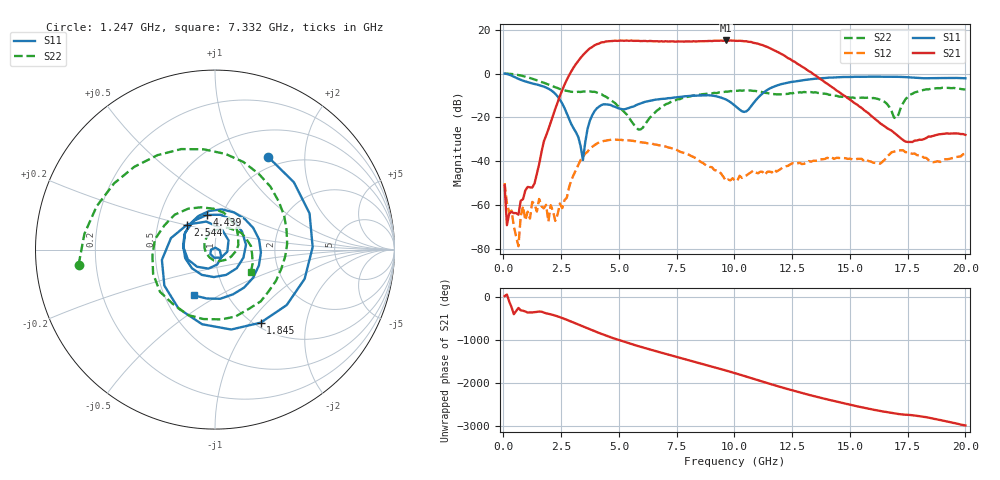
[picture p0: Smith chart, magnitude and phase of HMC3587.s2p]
! Analog Devices, Inc.
! Device:  HMC3587LP3BE
! Description:	HBT GAIN BLOCK MMIC AMPLIFIER, 4 - 10 GHz
! Conditions:	Vcc = 5.0 V
!  Idd = 45.8 mA
!  Pin = -20 dBm
!  Operating Temperature = +25C
! Engineering Evaluation unit (SN4) measured on PCB
! Measurements are referenced to PCB coaxial connectors with the exception of S21a(dB), for which the THRU CAL loss has been de-embedded.
! Freq(GHz)	S11a(dB)	S11p(deg)	S21a(dB)	S21p(deg)	S12a(dB)	S12p(deg)	S22a(dB)	S22p(deg)
# GHz S DB R 50
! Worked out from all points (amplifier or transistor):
!   201 points, 50 MHz to 20 GHz, reference 50 ohm
!   highest |S21| = 15.1 dB at 9.626 GHz (marker M1)
!   |S21| within 3 dB of that: 3.838 GHz to 11.43 GHz (7.595 GHz wide, 99.5 % of centre)
!   unconditionally stable (mu >= 1): start of sweep to end of sweep
!   at 3.342 GHz: K = 17.39, MAG = 7.8 dB, |S12| = -39.3 dB
!   at 10.03 GHz: K = 19.84, MAG = 15.9 dB, |S12| = -48.8 dB
!   at 20 GHz: K = 262.24, MAG = -22.9 dB, |S12| = -36.5 dB
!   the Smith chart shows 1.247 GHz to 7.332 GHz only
!   S11 on the Smith chart (normalised r, x): 1.247 GHz: 0.84, +1.35; 1.845 GHz: 1.07, -1.13; 2.544 GHz: 0.71, +0.21; 4.439 GHz: 0.85, +0.34; 7.332 GHz: 0.70, -0.39
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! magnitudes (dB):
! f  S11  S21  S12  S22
! 50 MHz  0.0  -51.0  -49.9  -0.1
! 149.8 MHz  -0.2  -69.1  -59.0  0.0
! 648.5 MHz  -2.4  -64.3  -78.6  -0.7
! 848 MHz  -3.2  -57.2  -60.4  -1.1
! 1.147 GHz  -4.2  -51.8  -66.0  -2.0
! 1.247 GHz  -4.5  -51.9  -58.4  -2.3
! 1.845 GHz  -6.4  -28.3  -59.8  -4.6
! 1.945 GHz  -6.9  -25.4  -67.4  -5.0
! 2.045 GHz  -7.5  -22.3  -59.9  -5.4
! 2.244 GHz  -9.2  -16.1  -67.1  -6.2
! 2.544 GHz  -13.6  -7.6  -61.3  -7.3
! 3.442 GHz  -39.4  8.4  -37.8  -8.2
! 3.741 GHz  -21.5  11.5  -34.2  -8.1
! 4.439 GHz  -14.0  14.6  -30.6  -10.5
! 5.835 GHz  -14.0  14.9  -31.1  -25.5
! 6.733 GHz  -11.7  14.6  -32.7  -16.2
! 7.332 GHz  -11.0  14.7  -34.2  -12.5
! 9.626 GHz  -11.8  15.1  -48.8  -8.2
! 10.03 GHz  -14.7  15.0  -48.8  -7.9
! 13.42 GHz  -2.4  -0.3  -39.7  -8.6
! 16.71 GHz  -1.4  -25.4  -36.8  -15.3
! 20 GHz  -2.1  -27.9  -36.5  -7.2
